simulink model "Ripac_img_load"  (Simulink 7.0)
settings: Solver=FixedStepDiscrete  StartTime=0.0  StopTime=row  RelTol=1e-3
PreLoadFcn:
  | [r,g,b]=Ripac_img_start('DSC_2750.resized.JPG');
  | 
  | col=r.signals.dimensions;
  | row=size(r.signals.values,1);
  | 
  | kernel = [-1 0 1; -2 0 2; -1 0 1];
InitFcn:
  | [r,g,b]=Ripac_img_start('DSC_2750.resized.JPG');
  | 
  | col=r.signals.dimensions;
  | row=size(r.signals.values,1);
  | 
  | kernel = [-1 0 1; -2 0 2; -1 0 1];
StopFcn:
  | obr_out=Ripac_img_stop(hrana,col);
  | 
  | obr2=int16((double(obr_out)).^(1/2));
  | 
  | figure, image(obr2); colormap('gray'), title('Final Edge Detected Image')
libraries: simulink x2, dspbuff3 x1

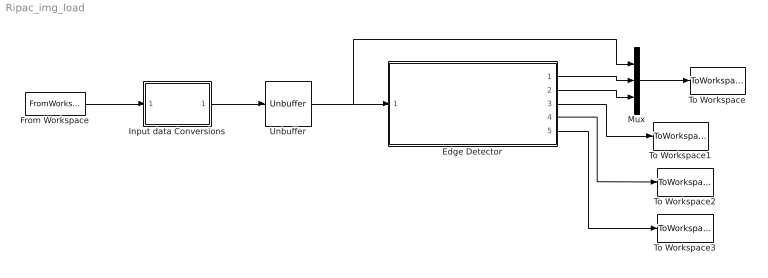
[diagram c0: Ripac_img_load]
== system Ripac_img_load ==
  Edge Detector : Subsystem
  From Workspace : FromWorkspace  VariableName=r  SampleTime=0  Interpolate=off  OutputAfterFinalValue=Setting to zero
  Input data Conversions : Subsystem
  Mux : Mux  Inputs=3
  To Workspace : ToWorkspace  VariableName=simout  SampleTime=-1  SaveFormat=Structure With Time
  To Workspace1 : ToWorkspace  VariableName=hrana  SampleTime=-1  SaveFormat=Structure With Time
  To Workspace2 : ToWorkspace  VariableName=hrana1  SampleTime=-1  SaveFormat=Structure With Time
  To Workspace3 : ToWorkspace  VariableName=hrana2  SampleTime=-1  SaveFormat=Structure With Time
  Unbuffer : dspbuff3/Unbuffer  ic=0
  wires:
  From Workspace/1 -> Input data Conversions/1(In)
  Unbuffer/1 -> Mux/1, Edge Detector/1(Row Input)
  Input data Conversions/1(Out) -> Unbuffer/1
  Edge Detector/3(Detector Out) -> To Workspace1/1
  Mux/1 -> To Workspace/1
  Edge Detector/1(Delay Line Out 1) -> Mux/2
  Edge Detector/2(Delay Line Out 2) -> Mux/3
  Edge Detector/4(Detector Out1) -> To Workspace2/1
  Edge Detector/5(Detector Out2) -> To Workspace3/1

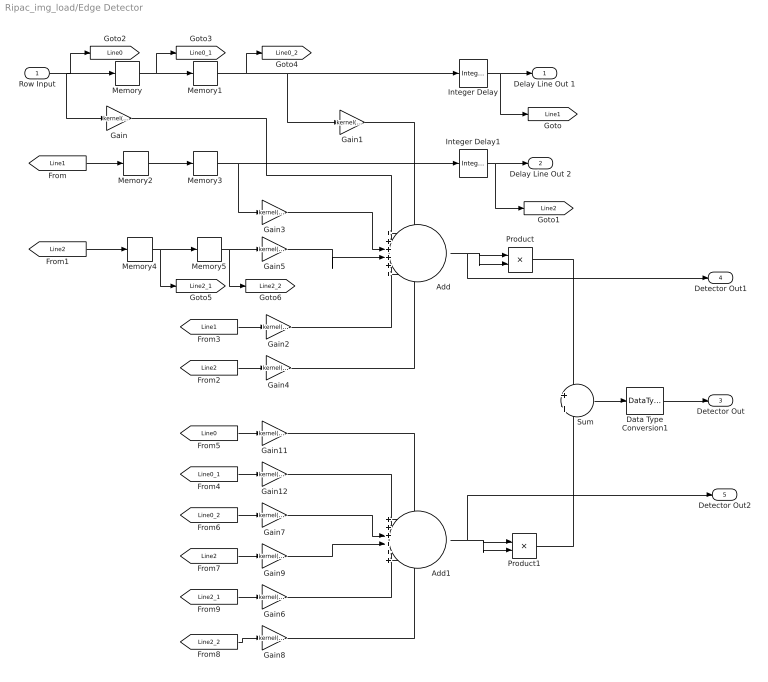
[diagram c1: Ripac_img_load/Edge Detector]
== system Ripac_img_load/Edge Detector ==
  Row Input : Inport
  Add : Sum  Inputs=++++++  OutDataType=sfix(16)  OutScaling=2^-10
  Add1 : Sum  Inputs=++++++  OutDataType=sfix(16)  OutScaling=2^-10
  Data Type Conversion1 : DataTypeConversion  OutDataTypeMode=int16  OutDataType=sfix(16)  OutScaling=2^0
  Gain : Gain  Gain=kernel(1,1)  ParameterDataType=sfix(16)  ParameterScaling=2^0  OutDataType=sfix(16)  OutScaling=2^0
  Gain1 : Gain  Gain=kernel(1,3)  ParameterDataType=sfix(16)  ParameterScaling=2^0  OutDataType=sfix(16)  OutScaling=2^0
  Gain11 : Gain  Gain=kernel(1,1)  ParameterDataType=sfix(16)  ParameterScaling=2^0  OutDataType=sfix(16)  OutScaling=2^0
  Gain12 : Gain  Gain=kernel(2,1)  ParameterDataType=sfix(16)  ParameterScaling=2^0  OutDataType=sfix(16)  OutScaling=2^0
  Gain2 : Gain  Gain=kernel(2,1)  ParameterDataType=sfix(16)  ParameterScaling=2^0  OutDataType=sfix(16)  OutScaling=2^0
  Gain3 : Gain  Gain=kernel(2,3)  ParameterDataType=sfix(16)  ParameterScaling=2^0  OutDataType=sfix(16)  OutScaling=2^0
  Gain4 : Gain  Gain=kernel(3,1)  ParameterDataType=sfix(16)  ParameterScaling=2^0  OutDataType=sfix(16)  OutScaling=2^0
  Gain5 : Gain  Gain=kernel(3,3)  ParameterDataType=sfix(16)  ParameterScaling=2^0  OutDataType=sfix(16)  OutScaling=2^0
  Gain6 : Gain  Gain=kernel(2,3)  ParameterDataType=sfix(16)  ParameterScaling=2^0  OutDataType=sfix(16)  OutScaling=2^0
  Gain7 : Gain  Gain=kernel(3,1)  ParameterDataType=sfix(16)  ParameterScaling=2^0  OutDataType=sfix(16)  OutScaling=2^0
  Gain8 : Gain  Gain=kernel(3,3)  ParameterDataType=sfix(16)  ParameterScaling=2^0  OutDataType=sfix(16)  OutScaling=2^0
  Gain9 : Gain  Gain=kernel(1,3)  ParameterDataType=sfix(16)  ParameterScaling=2^0  OutDataType=sfix(16)  OutScaling=2^0
  Integer Delay : simulink/Discrete/Integer Delay  vinit=0.0  samptime=-1  NumDelays=col
  Integer Delay1 : simulink/Discrete/Integer Delay  vinit=0.0  samptime=-1  NumDelays=col
  Memory{,1..5} (6 alike) : Memory
  Product : Product  OutDataTypeMode=double  OutDataType=sfix(16)  OutScaling=2^0
  Product1 : Product  OutDataTypeMode=double  OutDataType=sfix(16)  OutScaling=2^0
  Sum : Sum  Inputs=+|+  OutDataType=sfix(16)  OutScaling=2^0
  Delay Line Out 1 : Outport
  Delay Line Out 2 : Outport  Port=2
  Detector Out : Outport  Port=3
  Detector Out1 : Outport  Port=4
  Detector Out2 : Outport  Port=5
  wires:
  Integer Delay/1 -> Delay Line Out 1/1, [Line1]
  Memory/1 -> Memory1/1, [Line0_1]
  Memory1/1 -> Integer Delay/1, Gain1/1, [Line0_2]
  Memory2/1 -> Memory3/1
  Memory3/1 -> Gain3/1, Integer Delay1/1
  Memory4/1 -> Memory5/1, [Line2_1]
  Memory5/1 -> Gain5/1, [Line2_2]
  Integer Delay1/1 -> Delay Line Out 2/1, [Line2]
  Gain1/1 -> Add/1
  Gain4/1 -> Add/6
  Row Input/1 -> Memory/1, Gain/1, [Line0]
  [Line1] -> Memory2/1
  [Line2] -> Memory4/1
  [Line2] -> Gain4/1
  [Line1] -> Gain2/1
  Gain/1 -> Add/2
  Gain3/1 -> Add/3
  Gain5/1 -> Add/4
  Gain2/1 -> Add/5
  Gain11/1 -> Add1/1
  Gain8/1 -> Add1/6
  Add1/1 -> Product1/1, Product1/2, Detector Out2/1
  Gain12/1 -> Add1/2
  Gain7/1 -> Add1/3
  Gain9/1 -> Add1/4
  Gain6/1 -> Add1/5
  [Line0] -> Gain11/1
  [Line0_2] -> Gain7/1
  [Line0_1] -> Gain12/1
  [Line2] -> Gain9/1
  [Line2_1] -> Gain6/1
  [Line2_2] -> Gain8/1
  Add/1 -> Product/1, Product/2, Detector Out1/1
  Product/1 -> Sum/1
  Product1/1 -> Sum/2
  Sum/1 -> Data Type Conversion1/1
  Data Type Conversion1/1 -> Detector Out/1

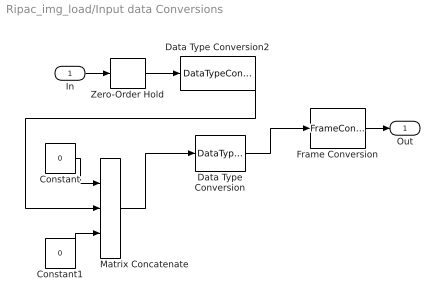
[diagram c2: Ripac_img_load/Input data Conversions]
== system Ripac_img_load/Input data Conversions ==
  In : Inport
  Constant : Constant  Value=0  OutDataType=sfix(16)  OutScaling=2^0
  Constant1 : Constant  Value=0  OutDataType=sfix(16)  OutScaling=2^0
  Data Type Conversion : DataTypeConversion  OutDataTypeMode=int16  OutDataType=sfix(16)  OutScaling=2^0
  Data Type Conversion2 : DataTypeConversion  OutDataTypeMode=double  OutDataType=sfix(16)  OutScaling=2^0
  Frame Conversion : FrameConversion
  Matrix Concatenate : Concatenate  NumInputs=3  Mode=Vector  ConcatenateDimension=2
  Zero-Order Hold : ZeroOrderHold
  Out : Outport
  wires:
  Zero-Order Hold/1 -> Data Type Conversion2/1
  Data Type Conversion/1 -> Frame Conversion/1
  Matrix Concatenate/1 -> Data Type Conversion/1
  Constant/1 -> Matrix Concatenate/1
  Constant1/1 -> Matrix Concatenate/3
  Data Type Conversion2/1 -> Matrix Concatenate/2
  In/1 -> Zero-Order Hold/1
  Frame Conversion/1 -> Out/1
